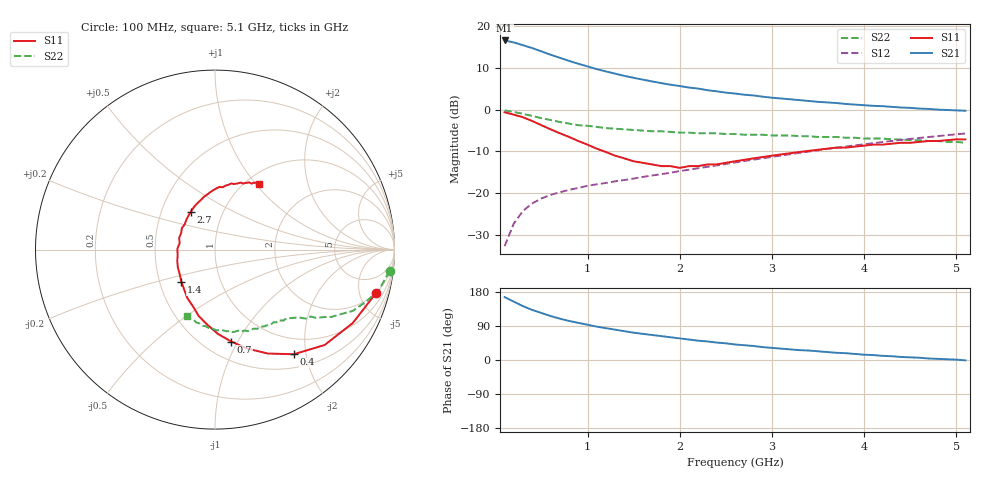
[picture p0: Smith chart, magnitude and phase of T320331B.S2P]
!AT-32033
!S PARAMETERS at Vce=1V  Ic=2mA.  LAST UPDATED 01-05-95
# ghz s ma r 50
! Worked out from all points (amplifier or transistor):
!   51 points, 100 MHz to 5.1 GHz, reference 50 ohm
!   highest |S21| = 16.6 dB at 100 MHz (marker M1)
!   |S21| within 3 dB of that: start of sweep to 546.4 MHz
!   unconditionally stable (mu >= 1): 1.625 GHz to 3.063 GHz
!   at 900 MHz: K = 0.74, MSG = 14.9 dB, |S12| = -18.8 dB
!   at 2.6 GHz: K = 1.03, MAG = 7.2 dB, |S12| = -12.7 dB
!   at 5.1 GHz: K = 0.91, MSG = 2.7 dB, |S12| = -5.7 dB
!   S11 on the Smith chart (normalised r, x): 100 MHz: 1.98, -7.05; 400 MHz: 0.71, -1.78; 700 MHz: 0.67, -0.94; 1.4 GHz: 0.65, -0.25; 2.7 GHz: 0.70, +0.31; 5.1 GHz: 1.15, +1.04
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0.1  0.93 -15.0  6.76 166.0  0.023 81.0  0.98 -7.0
0.2  0.87 -28.0  6.4 154.0  0.043 74.0  0.94 -14.0
0.3  0.81 -41.0  5.93 142.0  0.061 67.0  0.89 -19.0
0.4  0.73 -53.0  5.47 132.0  0.075 62.0  0.84 -24.0
0.5  0.65 -63.0  5 124.0  0.086 58.0  0.79 -27.0
0.6  0.58 -72.0  4.55 116.0  0.095 55.0  0.75 -30.0
0.7  0.52 -80.0  4.18 109.0  0.102 53.0  0.71 -32.0
0.8  0.47 -88.0  3.84 103.0  0.109 52.0  0.68 -34.0
0.9  0.42 -96.0  3.55 98.0  0.115 51.0  0.65 -35.0
1  0.38 -104.0  3.3 93.0  0.122 51.0  0.64 -37.0
1.1  0.34 -111.0  3.06 88.0  0.127 50.0  0.62 -38.0
1.4  0.26 -136.0  2.54 76.0  0.143 51.0  0.58 -41.0
1.5  0.24 -145.0  2.41 72.0  0.149 51.0  0.57 -42.0
1.8  0.21 -172.0  2.08 63.0  0.168 52.0  0.55 -46.0
2.2  0.21 154.0  1.79 51.0  0.198 52.0  0.52 -51.0
2.6  0.24 128.0  1.56 41.0  0.232 52.0  0.51 -57.0
2.7  0.25 123.0  1.51 39.0  0.242 52.0  0.5 -59.0
3  0.28 109.0  1.39 32.0  0.271 51.0  0.49 -64.0
3.5  0.33 92.0  1.24 23.0  0.325 48.0  0.47 -74.0
4  0.37 78.0  1.13 14.0  0.384 43.0  0.45 -85.0
4.3  0.39 71.0  1.08 10.0  0.42 40.0  0.44 -92.0
5.1  0.44 56.0  0.97 -1.0  0.517 30.0  0.4 -113.0
